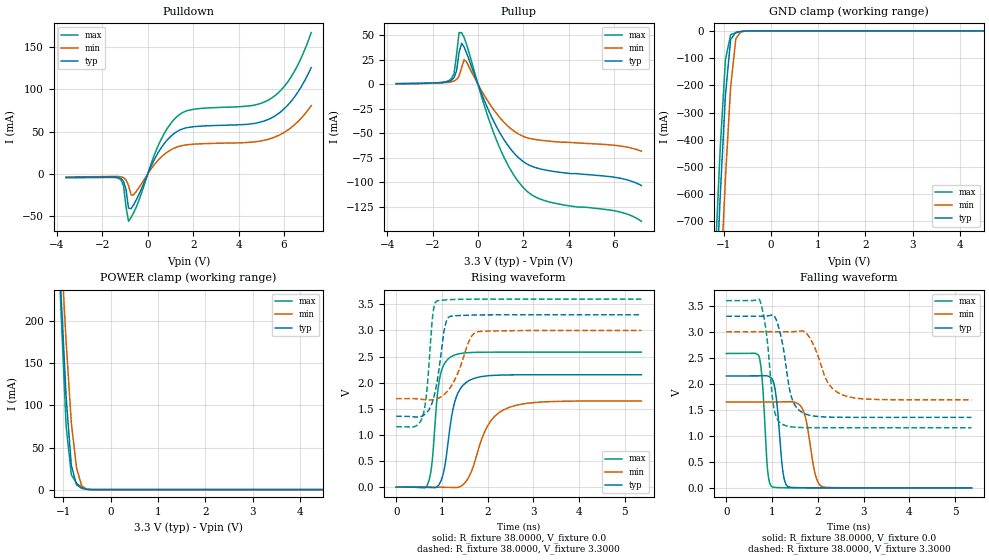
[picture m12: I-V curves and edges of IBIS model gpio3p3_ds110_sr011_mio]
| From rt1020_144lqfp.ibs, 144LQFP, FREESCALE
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[Model] gpio3p3_ds110_sr011_mio
|   Model gpio3p3_ds110_sr011_mio
| This model was characterised for following simulation conditions:
| External (pad) voltage:
|   - Typ: 3.3V,   - Min: 3.0V,   - Max: 3.6V
| Library cells for typ/min/max conditions are connected as defined below:
|  pad - External Pad
|  ipp_do - Core Input
|  ipp_obe - Output Buffer Enable
|  esd_boost - ovdd
|  ipp_dse0 - vssi
|  ipp_dse1 - vddi
|  ipp_dse2 - vddi
|  ipp_fsel0 - vddi
|  ipp_fsel1 - vddi
|  ipp_ina - ipp_ina
|  ipp_ind - ipp_ind
|  ipp_pwr_stable - vddi
|  ipp_sre - vssi
|  ovdd - ovdd
|  ovss - ovss
|  vddi - vddi
|  vssi - vssi
| All other pins connected to ground
Model_type I/O
Polarity   Non-Inverting
Enable   Active-High
Vinl =   0.9900V
Vinh =   2.3100V
Vmeas =  1.6500V
Cref =   0.0F
Rref =   38.0000
Vref =   1.6500V
C_comp   1.2179pF   1.1833pF   1.2636pF
|C_comp_pullup   0.6043pF   0.6190pF   0.5909pF
|C_comp_pulldown   0.5474pF   0.5788pF   0.5258pF
[Model Spec]
| variable   typ   min   max
Vinh   2.3100V   2.1000V   2.5200V
Vinl   0.9900V   0.9000V   1.0800V
S_overshoot_high   3.3000V   3.0000V   3.6000V
S_overshoot_low   0.0V   0.0V   0.0V
Vmeas   1.6500V   1.5000V   1.8000V
Vref   1.6500V   1.5000V   1.8000V
Cref   0.0F   0.0F   0.0F
Rref   38.0000   38.0000   38.0000
[Temperature Range]   25.0000   0.1050k   -20.0000
[Voltage Range]   3.3000V   3.0000V   3.6000V
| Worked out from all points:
|   slope of the pulldown table from 0 to 0.495 V, typ, clamps not added: 18.4 ohm
|   slope of the pullup table from 0 to 0.495 V, typ, clamps not added: 17.6 ohm
|   GND clamp passes 1 mA (typ) near -0.54 V on its own axis
|   POWER clamp passes 1 mA (typ) near -0.57 V on its own axis
|   rising waveform, R_fixture 38.0000, V_fixture 0.0: 20-80 % time 244ps typ, 458ps min, 157ps max; typ from 0 V to 2.15 V
|   rising waveform, R_fixture 38.0000, V_fixture 3.3000: 20-80 % time 204ps typ, 347ps min, 134ps max; typ from 1.36 V to 3.3 V
|   falling waveform, R_fixture 38.0000, V_fixture 0.0: 20-80 % time 126ps typ, 187ps min, 99.9ps max; typ from 2.15 V to 0 V
|   falling waveform, R_fixture 38.0000, V_fixture 3.3000: 20-80 % time 229ps typ, 364ps min, 165ps max; typ from 3.3 V to 1.36 V
[Pulldown]
|Voltage   I(typ)   I(min)   I(max)
-3.6V     -4.3mA     -3.7mA     -4.6mA
-1.29V    -4.333mA   -3.193mA   -5.198mA
-1.07V    -8.777mA   -4.485mA   -14.02mA
-960mV    -18.76mA   -7.185mA   -39.09mA
-850mV    -40.59mA   -13.79mA   -56.24mA
-630mV    -36.88mA   -25.09mA   -46.47mA
470mV     25.8mA     16.59mA    34.2mA
1.24V     49.32mA    31.28mA    66.64mA
1.9V      55.43mA    34.9mA     75.94mA
5.42V     65.92mA    41.89mA    89.15mA
6.3V      85.43mA    54.51mA    114.3mA
7.2V      126mA      80.78mA    167.4mA
[Pullup]
|Voltage   I(typ)   I(min)   I(max)
-3.6V     480uA      430uA      490uA
-1.27V    2.916mA    1.958mA    3.713mA
-1.05V    6.695mA    3.185mA    11mA
-940mV    13.85mA    4.743mA    30.4mA
-830mV    32.4mA     8.263mA    52.57mA
-720mV    41.6mA     16.53mA    52.38mA
-610mV    37.87mA    24.88mA    47.61mA
-500mV    31.75mA    22.65mA    40.51mA
820mV     -43.47mA   -29.95mA   -57.17mA
2.03V     -79.48mA   -53.58mA   -106.2mA
3.02V     -87.73mA   -57.84mA   -119.3mA
7.2V      -103.3mA   -68.29mA   -139.8mA
[GND_clamp]
|Voltage   I(typ)   I(min)   I(max)
-3.6V     -10.99A    -11.14A    -10.93A
-1.18V    -1.033A    -1.378A    -850.8mA
-1.07V    -607mA     -947.1mA   -431.4mA
-960mV    -236.8mA   -543mA     -106.4mA
-850mV    -31.63mA   -206.7mA   -14.18mA
-740mV    -5.424mA   -29mA      -7.092mA
-630mV    -2.275mA   -2.653mA   -3.283mA
-410mV    -62.05uA   -83.52uA   -82.04uA
7.2V      0A         0A         0A
[POWER_clamp]
|Voltage   I(typ)   I(min)   I(max)
-3.6V     3.491A     3.319A     3.949A
-1.16V    368.2mA    410.8mA    372.9mA
-1.05V    234.5mA    290.2mA    214.3mA
-940mV    110.2mA    175.6mA    75.85mA
-830mV    28.53mA    79.02mA    17.73mA
-720mV    5.671mA    25.66mA    7.515mA
-610mV    1.49mA     4.301mA    2.636mA
-500mV    198.2uA    300.8uA    424.4uA
-390mV    9.667uA    18.86uA    16.14uA
7.2V      0A         0A         0A
[Ramp]
| variable   typ   min   max
dV/dt_r  1.2910/0.2439n   0.9900/0.4576n   1.5507/0.1574n
dV/dt_f  1.1667/0.2293n   0.7844/0.3642n   1.4664/0.1651n
R_load = 38.0000
[Rising Waveform]
R_fixture= 38.0000
V_fixture= 0.0
V_fixture_min= 0.0
V_fixture_max= 0.0
|time   V(typ)   V(min)   V(max)
0s        2.972nV    2.696nV    31.46nV
688.7ps   -5.994mV   150.6uV    54.48mV
778.7ps   -10.43mV   -645.7uV   428.1mV
952ps     70.82mV    -2.728mV   2.093V
1.06ns    385.8mV    -4.323mV   2.37V
1.217ns   1.38V      -8.662mV   2.505V
1.526ns   2.001V     106mV      2.571V
1.985ns   2.13V      1.149V     2.584V
2.42ns    2.148V     1.509V     2.584V
5.36ns    2.152V     1.65V      2.585V
[Rising Waveform]
R_fixture= 38.0000
V_fixture= 3.3000
V_fixture_min= 3.0000
V_fixture_max= 3.6000
|time   V(typ)   V(min)   V(max)
0s        1.356V     1.693V     1.156V
419.1ps   1.341V     1.692V     1.164V
583.8ps   1.367V     1.677V     1.369V
674.5ps   1.432V     1.67V      1.883V
800.7ps   1.656V     1.673V     3.309V
888.6ps   1.991V     1.692V     3.564V
1.053ns   3.022V     1.775V     3.583V
1.177ns   3.268V     1.898V     3.59V
1.761ns   3.296V     2.97V      3.6V
5.36ns    3.3V       3V         3.6V
[Falling Waveform]
R_fixture= 38.0000
V_fixture= 0.0
V_fixture_min= 0.0
V_fixture_max= 0.0
|time   V(typ)   V(min)   V(max)
0s        2.152V     1.65V      2.585V
713ps     2.154V     1.65V      2.533V
795.2ps   2.157V     1.65V      1.954V
902.7ps   2.151V     1.65V      332.3mV
993.3ps   2.101V     1.651V     24.49mV
1.243ns   275.6mV    1.655V     2.367mV
1.354ns   21.77mV    1.659V     1.198mV
1.682ns   2.102mV    1.485V     249.5uV
2.099ns   336uV      23.52mV    95.11uV
5.36ns    1.592uV    14.56uV    1.84uV
[Falling Waveform]
R_fixture= 38.0000
V_fixture= 3.3000
V_fixture_min= 3.0000
V_fixture_max= 3.6000
|time   V(typ)   V(min)   V(max)
0s        3.3V       3V         3.6V
731.9ps   3.299V     3V         3.606V
874.1ps   3.304V     3V         2.99V
1.045ns   3.307V     3V         1.505V
1.226ns   2.786V     2.999V     1.223V
1.421ns   1.756V     3.002V     1.174V
1.724ns   1.423V     2.993V     1.159V
2.205ns   1.362V     2.046V     1.156V
2.547ns   1.357V     1.785V     1.156V
5.36ns    1.356V     1.693V     1.156V
